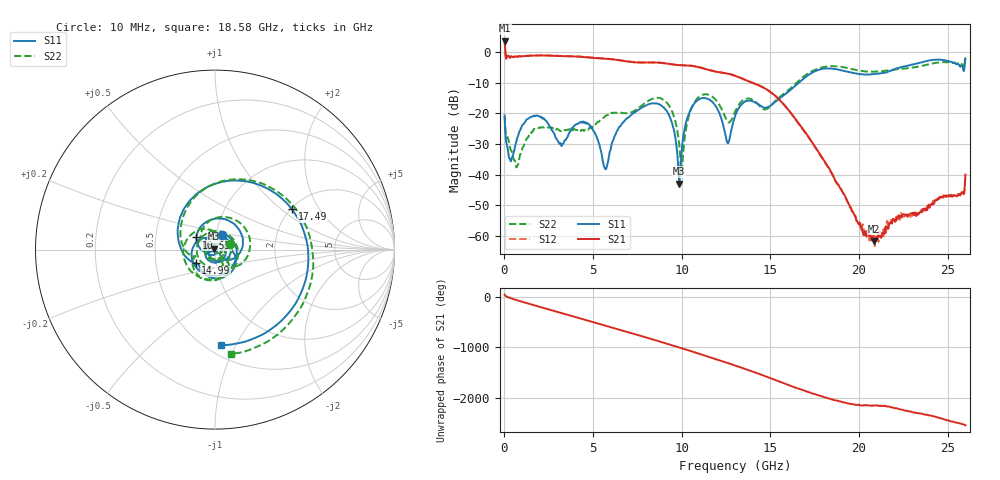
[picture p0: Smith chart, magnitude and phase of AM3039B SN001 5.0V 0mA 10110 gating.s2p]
!Agilent Technologies,E8364B,MY43040894,A.07.50.67
!Agilent E8364B: A.07.50.67
!Date: Tuesday, June 28, 2016 08:09:27
!Correction: S11(Full 2 Port(1,2))
!S21(Full 2 Port(1,2))
!S12(Full 2 Port(1,2))
!S22(Full 2 Port(1,2))
!S2P File: Measurements: S11, S21, S12, S22:
# Hz S  dB  R 50
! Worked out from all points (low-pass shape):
!   1601 points, 10 MHz to 26 GHz, reference 50 ohm
!   highest |S21| = 3.75 dB at 10 MHz (marker M1); lowest = -61.6 dB at 20.83 GHz (marker M2)
!   |S21| within 3 dB of the highest: start of sweep to 44 MHz
!   lowest |S11| = -42.9 dB at 9.854 GHz (marker M3), VSWR 1.01, Z = 49.5 + j0.519 ohm
!   |S11| at or under -10 dB: start of sweep to 16.6 GHz
!   |S22| runs from -39.0 to -1.2 dB; largest |S21 - S12| = 0.026
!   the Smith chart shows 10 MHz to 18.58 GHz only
!   S11 on the Smith chart (normalised r, x): 10 MHz: 1.07, +0.18; 10.55 GHz: 0.81, +0.11; 14.99 GHz: 0.80, -0.12; 17.49 GHz: 2.03, +1.19; 18.58 GHz: 0.59, -0.87
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1e7  -20.62 64.1  3.75 41.0  3.82 41.8  -21.08 21.0
7.409688e8  -27.76 115.1  -1.50 -73.9  -1.45 -73.7  -36.86 -178.4
1.715594e9  -20.96 20.0  -1.14 -173.7  -1.10 -173.4  -25.13 0.8
2.771438e9  -26.34 -122.5  -1.20 81.1  -1.12 81.3  -25.08 -168.1
4.347081e9  -22.98 -78.1  -1.54 -76.1  -1.51 -76.1  -25.42 -102.0
5.289219e9  -28.92 140.9  -2.00 -171.1  -1.95 -171.0  -22.73 59.6
6.182625e9  -27.86 -131.9  -2.40 97.8  -2.36 97.8  -19.70 -98.4
7.238469e9  -20.06 61.5  -3.27 -8.6  -3.22 -8.7  -19.49 70.7
8.684162e9  -16.89 -142.7  -3.43 -156.7  -3.37 -156.8  -14.93 -158.5
9.853712e9  -42.90 133.0  -4.24 79.7  -4.19 79.2  -29.69 62.1
1.055219e10  -18.15 146.8  -4.48 3.2  -4.43 2.7  -18.22 128.5
1.203038e10  -18.83 -26.1  -6.48 -161.4  -6.43 -162.3  -16.39 -37.8
1.3005e10  -20.95 -1.5  -7.69 84.3  -7.67 83.4  -19.45 -44.5
1.498674e10  -17.56 -144.8  -12.94 -163.4  -12.95 -164.7  -17.76 -163.9
1.734208e10  -6.75 42.9  -29.27 -102.0  -29.46 -103.2  -6.23 35.6
1.748828e10  -6.30 27.7  -30.59 -118.8  -30.75 -120.0  -5.82 21.9
1.857661e10  -5.46 -86.7  -40.76 124.7  -40.98 124.1  -4.61 -81.3
2.083449e10  -7.15 86.0  -61.62 16.7  -59.51 8.5  -6.40 96.3
2.167916e10  -6.28 27.4  -56.23 -2.9  -56.94 -5.9  -5.95 34.5
2.327105e10  -3.68 -93.3  -52.59 -129.9  -53.10 -129.3  -4.81 -82.4
2.437562e10  -2.43 176.5  -48.35 147.4  -48.25 144.7  -3.45 -167.2
2.6e10  -2.15 -10.2  -40.01 -16.3  -39.97 -17.4  -1.18 22.7
